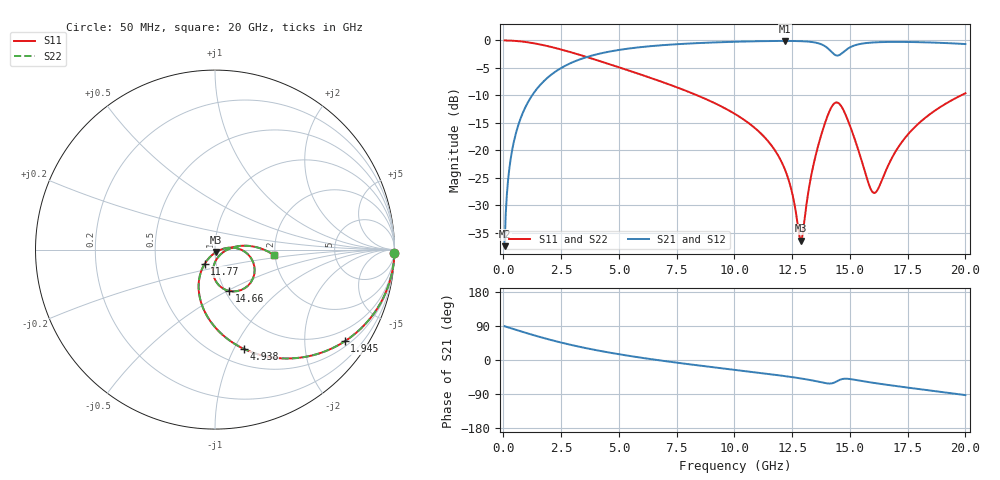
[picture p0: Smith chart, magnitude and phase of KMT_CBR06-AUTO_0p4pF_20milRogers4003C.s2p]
! Data measured by Modelithics Inc. support@modelithics.com 813-866-6335
! KEMET CBR06-AUTO 0.4pF, Pad Width= 0.851mm, Pad Length= 0.64mm, Pad Gap= 0.62mm, 20mil Rogers 4003C substrate Data, January 2022
# hz S ma R 50
! 2 Port Network Data from SP1.SP block
! freq  magS11  angS11  magS21  angS21  magS12  angS12  magS22  angS22
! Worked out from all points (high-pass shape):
!   401 points, 50 MHz to 20 GHz, reference 50 ohm
!   highest |S21| = -0.09 dB at 12.17 GHz (marker M1); lowest = -37.5 dB at 50 MHz (marker M2)
!   |S21| within 3 dB of the highest: 3.562 GHz to end of sweep
!   lowest |S11| = -36.5 dB at 12.87 GHz (marker M3), VSWR 1.03, Z = 50.7 - j1.36 ohm
!   |S11| at or under -10 dB: 8.388 GHz to 19.81 GHz (11.42 GHz wide, 81 % of centre)
!   |S22| runs from -36.5 to 0.0 dB; largest |S21 - S12| = 0
!   S11 on the Smith chart (normalised r, x): 50 MHz: open; 1.945 GHz: 0.64, -3.02; 4.938 GHz: 0.66, -1.09; 11.77 GHz: 0.88, -0.14; 14.66 GHz: 1.05, -0.51; 20 GHz: 1.98, -0.14
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5e7  0.9999 -1.0  0.01336 89.0  0.01336 89.0  0.9999 -1.0
2.99375e8  0.9968 -5.7  0.07977 84.2  0.07977 84.2  0.9968 -5.7
5.98625e8  0.9873 -11.4  0.1581 78.5  0.1581 78.5  0.9873 -11.4
1.14725e9  0.9556 -21.6  0.294 68.4  0.294 68.4  0.9556 -21.6
1.94525e9  0.8849 -35.3  0.4645 54.6  0.4645 54.6  0.8849 -35.3
3.391625e9  0.7295 -56.3  0.6821 33.6  0.6821 33.6  0.7295 -56.3
4.93775e9  0.5752 -73.9  0.8156 15.9  0.8156 15.9  0.5752 -73.9
6.73325e9  0.4288 -90.4  0.9006 -0.7  0.9006 -0.7  0.4288 -90.4
1.0025e10  0.2139 -115.2  0.9731 -26.1  0.9731 -26.1  0.2139 -115.2
1.177062e10  0.09856 -125.9  0.9891 -39.2  0.9891 -39.2  0.09856 -125.9
1.216962e10  0.0681 -126.2  0.99 -42.4  0.99 -42.4  0.0681 -126.2
1.286788e10  0.01497 -63.3  0.9851 -48.6  0.9851 -48.6  0.01497 -63.3
1.296762e10  0.01793 -26.5  0.983 -49.6  0.983 -49.6  0.01793 -26.5
1.336662e10  0.06502 7.9  0.9671 -53.9  0.9671 -53.9  0.06502 7.9
1.411475e10  0.2264 -19.1  0.822 -62.1  0.822 -62.1  0.2264 -19.1
1.466338e10  0.2443 -70.8  0.767 -50.2  0.767 -50.2  0.2443 -70.8
1.511225e10  0.1444 -93.0  0.8872 -51.2  0.8872 -51.2  0.1444 -93.0
1.596012e10  0.04207 -57.9  0.9574 -59.8  0.9574 -59.8  0.04207 -57.9
1.62095e10  0.04406 -25.7  0.9636 -62.0  0.9636 -62.0  0.04406 -25.7
1.670825e10  0.07647 2.6  0.9694 -66.3  0.9694 -66.3  0.07647 2.6
1.795512e10  0.1737 7.2  0.965 -76.4  0.965 -76.4  0.1737 7.2
2e10  0.3307 -5.4  0.9272 -92.6  0.9272 -92.6  0.3307 -5.4
